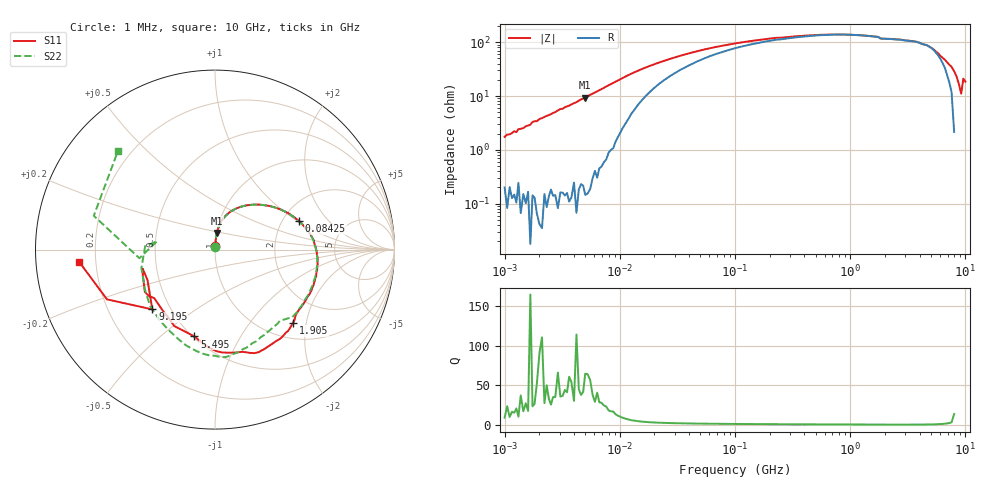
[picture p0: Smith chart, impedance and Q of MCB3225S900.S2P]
!Agilent Technologies,E5071C,MY46111244,A.11.31
!Date: Thu May 09 18:33:09 2019
!Data & Calibration Information:
!Freq	S11:SOLT2(ON)	S21:SOLT2(ON)	S12:SOLT2(ON)	S22:SOLT2(ON)
# Hz S dB R 50
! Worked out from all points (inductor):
!   201 points, 1 MHz to 10 GHz, reference 50 ohm
!   read as one part in series: L = 283 nH near 1.053 MHz
!   highest Q = 56.7 at 5.012 MHz (marker M1), where L = 297 nH
!   self-resonance near 1.179 GHz
!   S11 on the Smith chart (normalised r, x): 1 MHz: 1.00, +0.04; 84.25 MHz: 2.46, +1.03; 1.905 GHz: 1.32, -1.68; 5.495 GHz: 0.51, -0.65; 9.195 GHz: 0.40, -0.35; 10 GHz: 0.14, -0.05
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1000000  -34.76 83.5  -0.02 -1.1  -0.03 -0.8  -35.21 83.4
4810209  -21.12 83.2  -0.06 -5.2  -0.05 -5.1  -21.09 84.1
5011872  -20.68 84.1  -0.04 -5.4  -0.06 -5.3  -20.66 83.3
1.212171e7  -12.69 67.3  -0.57 -13.5  -0.58 -13.5  -12.68 67.2
2.206931e7  -9.37 47.6  -1.80 -18.5  -1.82 -18.5  -9.38 47.6
8.425348e7  -6.11 18.6  -5.01 -19.2  -5.02 -19.2  -6.11 18.5
1.047129e8  -5.85 15.4  -5.44 -18.4  -5.44 -18.4  -5.85 15.3
4.810209e8  -4.83 -5.2  -7.42 -14.0  -7.43 -14.0  -4.85 -5.5
1.213756e9  -4.70 -25.5  -7.74 -17.7  -7.74 -17.7  -4.79 -27.0
1.75212e9  -4.76 -38.8  -7.76 -23.6  -7.79 -23.6  -4.85 -41.0
1.905461e9  -4.49 -43.3  -7.60 -26.9  -7.59 -26.9  -5.36 -49.7
2.206931e9  -4.31 -48.1  -7.78 -29.7  -7.79 -29.7  -5.29 -56.2
3.630781e9  -4.19 -69.1  -8.31 -43.0  -8.32 -43.0  -4.66 -77.1
4.83488e9  -4.94 -89.1  -8.27 -57.8  -8.25 -57.8  -4.49 -88.3
5.495409e9  -6.07 -103.4  -8.00 -69.5  -7.99 -69.5  -4.67 -96.7
6.952868e9  -7.27 -141.4  -7.34 -98.7  -7.38 -98.5  -6.03 -128.3
7.585776e9  -6.82 -148.9  -6.98 -113.0  -6.97 -113.0  -6.95 -150.1
7.988146e9  -7.45 -161.9  -6.76 -125.5  -6.76 -125.4  -7.47 -165.8
8.792888e9  -7.70 -155.8  -5.97 -161.4  -6.00 -161.2  -9.77 171.6
9.195259e9  -6.33 -136.3  -6.54 159.8  -6.56 159.8  -7.45 -173.5
9.597629e9  -3.57 -155.3  -10.36 110.5  -10.39 110.4  -3.08 164.4
1e10  -2.40 -174.7  -11.52 62.8  -11.54 62.6  -2.27 134.7
